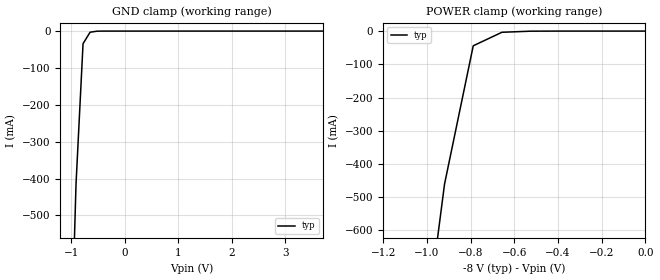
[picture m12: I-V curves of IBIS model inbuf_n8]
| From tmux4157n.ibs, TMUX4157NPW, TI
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| inbuf_n8
[Model]   inbuf_n8
Model_type   Input
Vinl = 0.8
Vinh = 1.35
|   typ   min   max
C_comp   6.976543e-12   NA   NA
[Voltage Range]   -8   NA   NA
[Temperature Range]   27   NA   NA
[Power Clamp Reference]   -8   NA   NA
[GND Clamp Reference]   0   NA   NA
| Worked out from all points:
|   GND clamp passes 1 mA (typ) near -0.55 V on its own axis
|   POWER clamp passes 1 mA (typ) near -0.55 V on its own axis
[GND Clamp]
|   Voltage   I(typ)   I(min)   I(max)
-8V       -30.34A    NA         NA
-1.04V    -1.073A    NA         NA
-909.1mV  -414.9mA   NA         NA
-777.8mV  -34.15mA   NA         NA
-646.5mV  -3.104mA   NA         NA
-383.8mV  -3.239uA   NA         NA
5V        2.234uA    NA         NA
[POWER Clamp]
|   Voltage   I(typ)   I(min)   I(max)
-13V      -49.45A    NA         NA
-1.051V   -1.128A    NA         NA
-919.2mV  -460.6mA   NA         NA
-787.9mV  -44.23mA   NA         NA
-656.6mV  -3.592mA   NA         NA
-525.3mV  -291.6uA   NA         NA
0V        161.9pA    NA         NA
